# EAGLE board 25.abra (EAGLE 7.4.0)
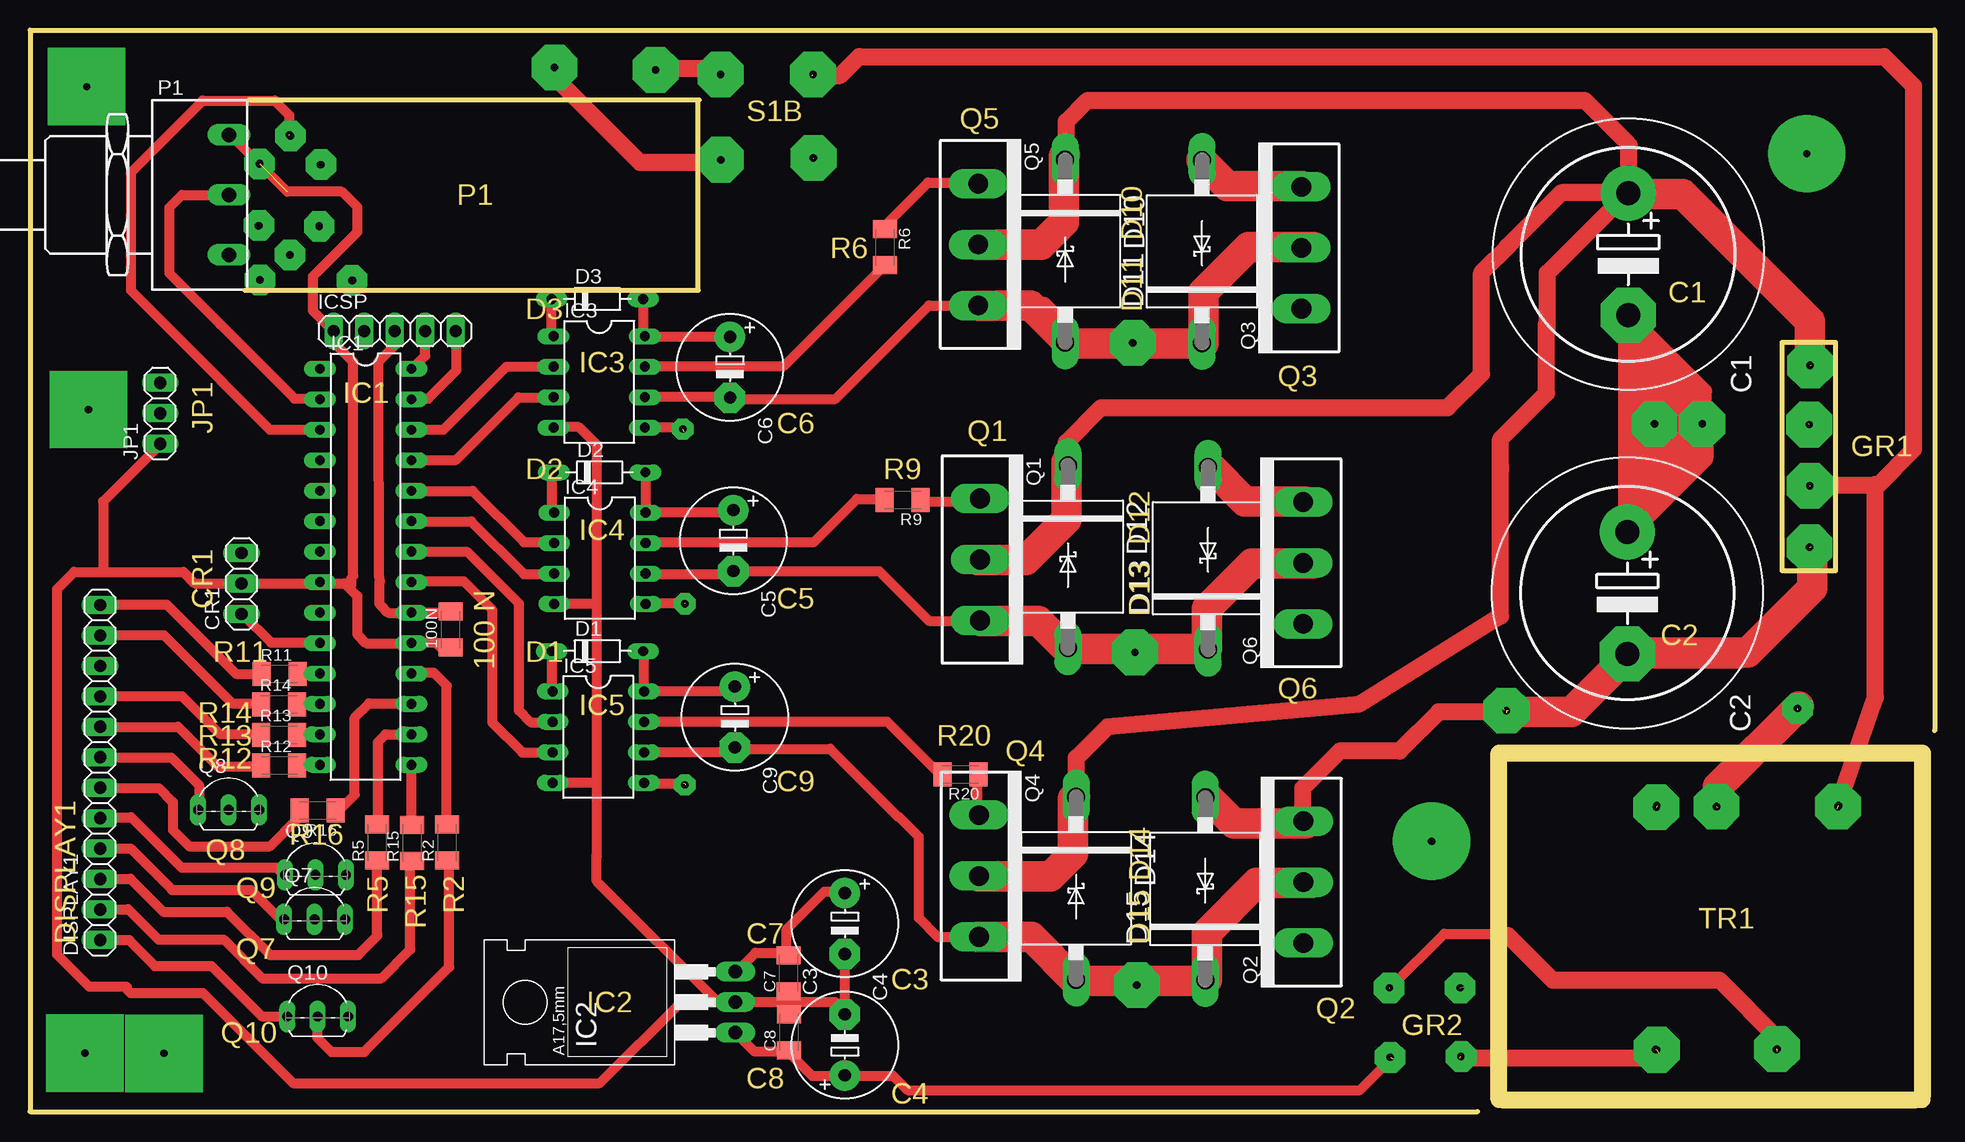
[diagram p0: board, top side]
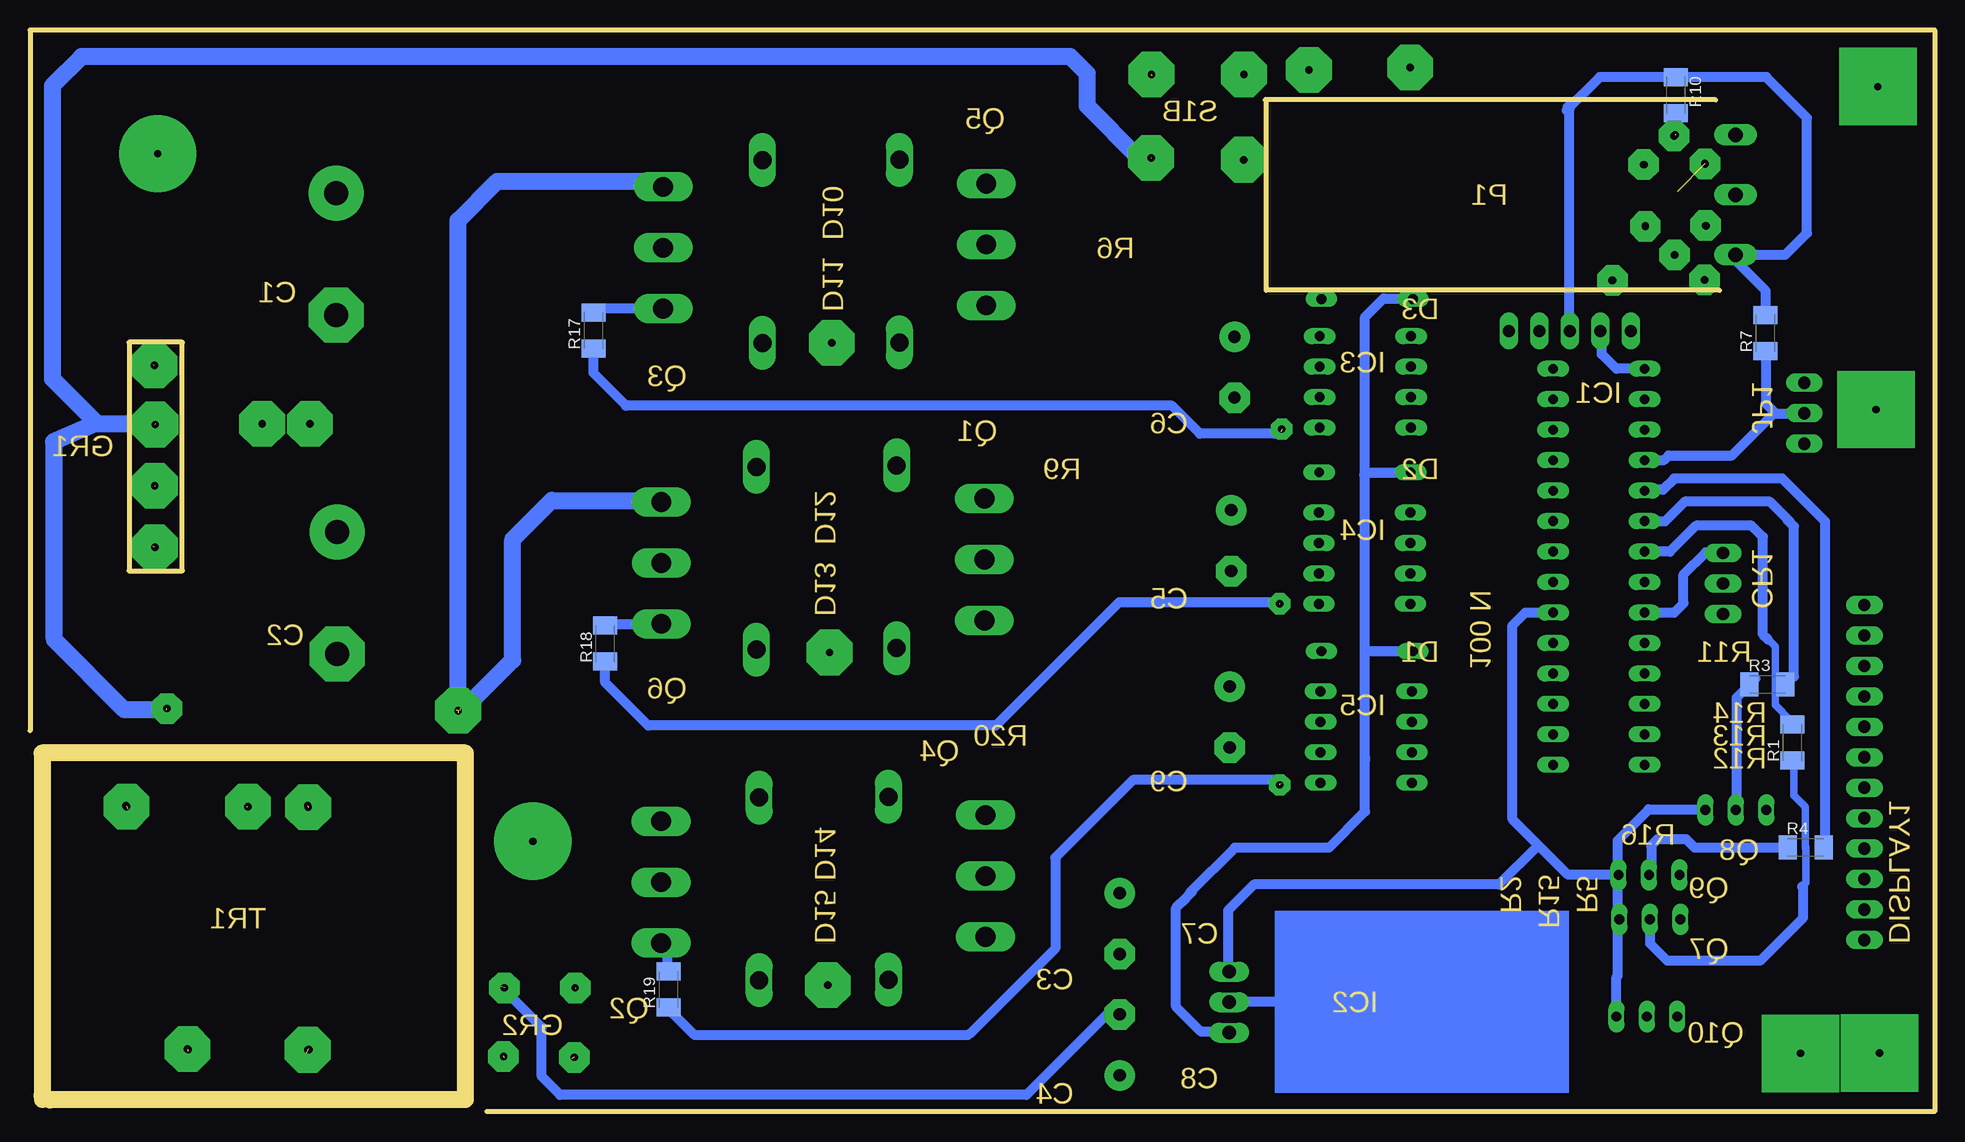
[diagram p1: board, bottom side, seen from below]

Size 158.75 x 90.17 mm. Coordinates in mm from the lower left corner, seen from the top.
Outline: 122.45,0.99 122.45,29.9 157.73,29.9 157.73,1.32
Outline: 122.66,0.99 157.07,0.96 157.71,1.02
Outline: 17.91,68.48 55.7,68.48 55.7,84.25
Outline: 18.26,84.35 55.8,84.35
Outline: 158.75,31.75 158.75,90.17 0,90.17 0,0 120.65,0
Outline: 146.05,64.14 150.5,64.14 150.5,45.09 146.05,45.09 146.05,64.14
Copper layers (1*16): Top 0.035mm / dielectric 1.5mm / Bottom 0.035mm
Design rules "default": minimum track width 10mil, minimum drill 24mil, track to track 8mil, track to pad 8mil, pad to pad 8mil, via to via 8mil, smd to smd 8mil, copper to edge 40mil, drill to drill 8mil, minimum pad ring 10mil, minimum via ring 8mil, stop-mask expansion 4mil, vias tented up to drill 0mil, thermal gap 10mil

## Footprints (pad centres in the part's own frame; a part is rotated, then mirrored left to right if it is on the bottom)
C1206K = smd 1.5 x 2: 1 -1.5,0; 2 1.5,0
EB22,5D = drill 2.007 pad 4.597: + -5.08,0 | drill 2.007 pad 4.597 octagon: - 5.08,0
E5-8,5 = drill 1.016 pad 2.54: + -2.54,0 | drill 1.016 pad 2.54 octagon: - 2.54,0
1X03 = drill 1.016 long: 1 -2.54,0; 2 0,0; 3 2.54,0
D-7.5 = drill 0.813 long: A 3.81,0; C -3.81,0
P6T15 = drill 1.499 long: A 7.62,0; C -7.62,0
1X12 = drill 1.016 long: 1 -13.97,0; 2 -11.43,0; 3 -8.89,0; 4 -6.35,0; 5 -3.81,0; 6 -1.27,0; 7 1.27,0; 8 3.81,0; 9 6.35,0; 10 8.89,0; 11 11.43,0; 12 13.97,0
DIL28-3 = drill 0.813 long: 1 -16.51,-3.81; 2 -13.97,-3.81; 3 -11.43,-3.81; 4 -8.89,-3.81; 5 -6.35,-3.81; 6 -3.81,-3.81; 7 -1.27,-3.81; 8 1.27,-3.81; 9 3.81,-3.81; 10 6.35,-3.81; 11 8.89,-3.81; 12 11.43,-3.81; 13 13.97,-3.81; 14 16.51,-3.81; 15 16.51,3.81; 16 13.97,3.81; 17 11.43,3.81; 18 8.89,3.81; 19 6.35,3.81; 20 3.81,3.81; 21 1.27,3.81; 22 -1.27,3.81; 23 -3.81,3.81; 24 -6.35,3.81; 25 -8.89,3.81; 26 -11.43,3.81; 27 -13.97,3.81; 28 -16.51,3.81
TO220 = drill 1.118 long: 1 -2.54,-10.16; 2 0,-10.16; 3 2.54,-10.16
DIL08 = drill 0.813 long: 1 -3.81,-3.81; 2 -1.27,-3.81; 3 1.27,-3.81; 4 3.81,-3.81; 5 3.81,3.81; 6 1.27,3.81; 7 -1.27,3.81; 8 -3.81,3.81
1X05 = drill 1.016 long: 1 -5.08,0; 2 -2.54,0; 3 0,0; 4 2.54,0; 5 5.08,0
PC16S = drill 1.2 long: 1A -5,6.5; 1E 5,6.5; 1S 0,6.5
TO258AA-V = drill 1.651 long: 1-D -5.08,0; 2-S 0,0; 3-G 5.08,0
TO92-BCE = drill 0.813 long: B 2.54,0; C 0,0; E -2.54,0

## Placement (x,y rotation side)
100N  [C1206K]  35.05,40.18 90 top
C1  [EB22,5D]  133.22,71.48 270 top
C2  [EB22,5D]  133.15,43.23 270 top
C3  [E5-8,5]  67.92,5.56 90 top
C4  [E5-8,5]  67.92,15.67 270 top
C5  [E5-8,5]  58.62,47.6 270 top
C6  [E5-8,5]  58.34,62.05 270 top
C7  [C1206K]  63.25,11.53 90 top
C8  [C1206K]  63.27,6.6 90 top
C9  [E5-8,5]  58.75,32.89 270 top
CR1  [1X03]  17.63,44.02 90 top
D1  [D-7.5]  47.29,38.38 0 top
D2  [D-7.5]  47.47,53.29 0 top
D3  [D-7.5]  47.29,67.74 0 top
D10  [P6T15]  86.28,71.73 270 top
D11  [P6T15]  97.69,71.7 90 top
D12  [P6T15]  86.51,46.25 270 top
D13  [P6T15]  98.2,46.13 90 top
D14  [P6T15]  87.2,18.62 270 top
D15  [P6T15]  97.97,18.57 90 top
DISPLAY1  [1X12]  5.84,28.27 90 top
IC1  [DIL28-3]  27.97,45.41 270 top
IC2  [TO220]  48.64,9.12 90 top
IC3  [DIL08]  47.45,60.83 270 top
IC4  [DIL08]  47.5,46.13 270 top
IC5  [DIL08]  47.37,31.22 270 top
ICSP  [1X05]  30.4,65.07 0 top
JP1  [1X03]  10.85,58.22 90 top
P1  [PC16S]  10.08,76.43 270 top
Q1  [TO258AA-V]  79.2,46.02 270 top
Q2  [TO258AA-V]  106.15,19.13 90 top
Q3  [TO258AA-V]  105.97,72.01 90 top
Q4  [TO258AA-V]  79.1,19.63 270 top
Q5  [TO258AA-V]  79.04,72.29 270 top
Q6  [TO258AA-V]  106.12,45.75 90 top
Q7  [TO92-BCE]  23.72,16.03 0 top
Q8  [TO92-BCE]  16.56,25.15 0 top
Q9  [TO92-BCE]  23.8,19.74 0 top
Q10  [TO92-BCE]  23.98,7.92 0 top
R1  [C1206K]  11.84,30.76 90 bottom
R2  [C1206K]  34.77,22.43 90 top
R3  [C1206K]  13.92,35.61 0 bottom
R4  [C1206K]  10.74,22.02 0 bottom
R5  [C1206K]  28.96,22.43 90 top
R6  [C1206K]  71.27,72.06 270 top
R7  [C1206K]  14.1,64.9 90 bottom
R9  [C1206K]  72.75,51 180 top
R10  [C1206K]  21.56,84.73 270 bottom
R11  [C1206K]  20.8,36.47 0 top
R12  [C1206K]  20.78,28.85 0 top
R13  [C1206K]  20.75,31.42 0 top
R14  [C1206K]  20.75,33.96 0 top
R15  [C1206K]  31.85,22.4 90 top
R16  [C1206K]  23.98,25.1 180 top
R17  [C1206K]  111.79,65.13 90 bottom
R18  [C1206K]  110.79,39.01 90 bottom
R19  [C1206K]  105.54,10.19 90 bottom
R20  [C1206K]  77.55,28.12 180 top

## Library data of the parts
100N C7 C8 Q1-Q6 R1-R7 R9-R20 = ref-packages
C1-C6 C9 = rcl
CR1 DISPLAY1 ICSP JP1 = pinhead
D1-D3 D10-D15 = diode
IC1 IC3-IC5 = 40xx
IC2 = mc33269
P1 = piher
Q7-Q10 = transistor

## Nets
S$53: ICSP.4
S$101: D1.C
S$111: Q3.2-S
S$112: D10.A
S$140: C5.-

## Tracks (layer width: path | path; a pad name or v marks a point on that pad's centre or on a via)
C5
  Top 0.813: 51.31,47.5 65.35,47.5 68.94,51.08 70.99,51.08 71.09,50.98
D1
  Top 0.813: 43.71,57.05 45.77,57.05 47.27,55.55 47.27,21.29
Q1
  Top 0.813: 79.35,77.44 74.85,77.44 71.09,73.69
S$1  (via drill 0.61 pad 6.45)
  other vias: 4.72,85.45
S$2  (via drill 0.61 pad 6.45)
  other vias: 4.57,4.88
S$3  (via drill 0.61 pad 3.81)  (1 unrouted)
  Top 1.422: 148.46,47.12 148.46,43.56 142.54,37.64 132.99,37.64 132.72,37.92
  other vias: 148.34,47.04
S$4
  Top 0.813: 5.84,42.27 11.4,42.27 17.17,36.5 18.95,36.5 19,36.45 | 19,36.45 19.15,36.45 | 19,36.45 18.41,36.45
S$5
  Top 0.813: 5.87,39.73 11.15,39.73 16.84,34.04 19.05,34.04
S$6
  Top 0.813: 5.84,34.65 12.65,34.65 15.8,31.5 18.82,31.5 18.9,31.42
S$7
  Top 0.813: 18.34,28.78 19.15,28.78
S$8
  Top 0.813: 24.16,39.09 20.09,39.09 17.65,41.53
S$9
  Bottom 0.813: 24.18,41.58 21.72,41.58 20.93,42.37 20.93,44.76 19.07,46.61 18.03,46.61 17.98,46.56
S$10
  Bottom 0.813: 34.65,4.39 34.75,4.29
S$11
  Top 0.813: 5.87,19.41 8.36,19.41 11.1,16.66 16.41,16.66 20.02,13.06 27.36,13.06 28.96,14.66
S$12
  Top 0.813: 5.84,24.54 8.43,24.54 12.62,20.34 20.55,20.34 21.29,19.61
S$13
  Top 0.813: 5.87,32.08 12.34,32.08 15.65,28.78 19.28,28.78
S$14
  Top 0.813: 5.77,14.28 8.28,14.28 10.03,12.52
S$15
  Top 0.813: 5.87,29.52 11.79,29.52 14.1,27.2 14.1,25.22 13.99,25.12
S$16
  Top 0.813: 5.82,26.98 10.72,26.98 11.91,25.78 11.91,23.47 13.26,22.12 20.02,22.12 22.28,24.38
S$17
  Top 0.813: 31.83,34.04 28.27,34.04 27.08,32.84 27.08,26.42 25.78,25.12
S$18
  Top 0.813: 31.83,31.45 29.64,31.45 29.01,30.81 29.01,23.93
S$19
  Top 0.813: 31.83,28.96 31.83,23.8 31.88,23.75
S$20
  Top 0.813: 34.75,23.98 34.75,35.51 33.68,36.58 31.95,36.58 31.77,36.4
S$21
  Top 0.813: 5.77,21.92 8.38,21.92 11.84,18.47 18.41,18.47 20.88,16
S$22
  Top 0.813: 29.06,20.78 28.96,20.68 28.96,14.78
S$23
  Top 0.813: 5.87,16.87 8.18,16.87 10.69,14.35 16.13,14.35 19.36,11.12 29.31,11.12 31.7,13.51
S$24
  Top 0.813: 31.77,20.42 31.7,20.34 31.7,13.54
S$25
  Top 0.813: 21.44,7.95 19.3,7.95 15.11,12.14 10.39,12.14 9.98,12.55
S$26
  Top 0.813: 23.98,7.95 23.98,6.12 25.12,4.98 27.86,4.98 34.95,12.06 34.95,20.5 34.52,20.93
S$27
  Top 0.813: 58.88,9.12 54.25,9.12 47.5,2.36 21.92,2.36 14.4,9.88 8.36,9.88 7.8,10.44 | 17.6,44.04 13.74,44.04 12.8,44.98 3.68,44.98 2.26,43.56 2.26,13.08 4.9,10.44 7.8,10.44 | 17.6,44.04 17.68,44.04 | 7.8,10.44 8,10.44 8.08,10.36 | 31.8,39.04 28.04,39.04 27.28,39.8 27.28,43 26.24,44.04 24.18,44.04 | 24.18,44.04 23.98,44.04 | 17.6,44.04 24.18,44.04
S$28
  Top 0.813: 31.7,39.12 33.81,39.12 34.27,38.66
S$29
  Top 0.813: 17.42,46.63 17.45,46.66
S$30
  Bottom 0.813: 31.85,41.6 34.11,41.6 35.18,40.54 35.18,24.36 30.56,19.74 26.52,19.74 26.42,19.84 | 19.13,25.2 23.82,25.2 26.42,22.61 26.42,19.84 | 26.67,7.72 26.52,7.87 26.52,11.2 26.42,11.3 26.42,19.84
S$31
  Bottom 0.813: 52.81,9.14 58.9,9.14
S$32  (via drill 0.61 pad 6.45)
  other vias: 11.18,4.85
S$33
  Top 0.813: 58.85,9.14 63.2,9.14 | 63.2,9.14 63.93,9.14 | 63.2,9.14 67.13,9.14 68.22,8.05
S$34
  Top 0.813: 63.32,5.03 60.35,5.03 58.78,6.6
S$35
  Top 0.813: 63.25,13.23 60.48,13.23 58.95,11.71
S$36
  Top 0.813: 67.92,7.92 67.92,13.11
S$37
  Top 0.813: 67.92,2.97 65.2,2.97 63.32,4.85
S$38
  Top 0.813: 67.92,18.34 66.22,18.34 63.07,15.19 63.07,13.61 63.32,13.36
S$39
  Bottom 0.813: 58.88,11.58 58.88,16.76 56.72,18.92 36.3,18.92 33.2,22.02
S$40
  Bottom 0.813: 24.56,43.99 24.51,44.04 24.28,44.04 24.36,44.12
S$41
  Bottom 0.813: 12.39,22 19.99,22 20.7,22.71 23.09,22.71 23.62,22.17 23.62,19.66 23.8,19.48
S$42
  Top 0.813: 31.7,41.6 34.8,41.6
S$43
  Bottom 0.813: 24.16,46.69 22.05,46.69 19.89,48.84 15.27,48.84 14.33,47.9
S$44
  Bottom 0.813: 24.21,49.2 22.48,49.2 20.83,50.85 13.74,50.85 11.99,49.1
S$45
  Bottom 0.813: 24.21,51.84 22.63,51.84 21.69,52.78 12.7,52.78 9.12,49.2 9.12,46.46 | 9.12,22.05 9.12,46.46 | 9.12,46.46 9.12,46.69
S$46
  Bottom 0.813: 16.48,25.15 16.48,34.52 14.91,36.09
S$47
  Bottom 0.813: 11.71,36.27 11.71,48.79 12.29,49.38
S$48
  Bottom 0.813: 23.7,16.08 23.7,13.99 22.28,12.57 14.53,12.57 10.95,16.15 10.95,18.67 11.05,18.77
S$49
  Bottom 0.61: 10.77,22 10.77,25.4 11.71,26.34 11.71,28.8 11.81,28.91
S$50
  Bottom 0.61: 10.74,22.07 10.74,19.05 11.02,18.77
S$51
  Bottom 0.61: 13.28,37.03 13.28,37.06 | 13.28,37.03 13.28,33.88 11.96,32.56 | 13.28,37.03 13.28,38.79 14.05,39.55
S$52
  Bottom 0.813: 14.3,47.93 14.3,39.78 13.87,39.34
S$53
  Top 0.813: ICSP.4 32.94,63.02 31.77,61.85
S$54
  Top 0.813: 31.65,59.44 33.2,59.44 35.56,61.8 35.56,65.05 35.43,65.18
S$55
  Top 0.813: 31.95,59.46 31.85,59.36
S$56
  Top 0.813: 31.8,41.58 29.87,41.58 29.13,42.32 29.13,44.15
S$57
  Top 0.813: 29.08,60.55 29.11,44.53 29.16,44.17
S$58
  Bottom 0.813: 24.36,44.17 24.31,44.12
S$59
  Top 0.813: 26.77,43.92 26.77,44.48 26.95,44.65 26.95,62.48 25.2,64.24
S$60  (via drill 0.61 pad 1.78, 0.61 pad 2.54)  (2 unrouted)
  Top 0.813: 21.61,81.38 21.61,83.06 20.4,84.28 14.38,84.28 8.43,78.33 8.43,68.45 16.05,60.83
  Bottom 0.813: 21.57,83.08 21.57,81.46 21.54,81.43
  other vias: 21.62,81.43 21.72,81.33
S$61  (via drill 0.61 pad 1.78, 0.61 pad 2.54)
  other vias: 21.67,71.4 21.67,71.42
S$62  (via drill 0.61 pad 1.78, 0.61 pad 2.54)
  other vias: 19.18,69.32 19.18,69.34
S$63  (via drill 0.61 pad 1.78, 0.61 pad 2.54)  (1 unrouted)
  Top 0.813: 16.56,81.43 16.69,81.43 v19.13,78.99 21.44,76.68 26.01,76.68 27.3,75.39 27.3,73.36 23.6,69.65 23.6,66.75 25.38,64.97
  other vias: 19.15,79.04
S$64  (via drill 0.61 pad 1.78, 0.61 pad 2.54)
  other vias: 24.21,78.94 24.26,78.94
S$65  (via drill 0.61 pad 1.78, 0.61 pad 2.54)
  other vias: 24.1,73.84 24.1,73.79
S$66  (via drill 0.61 pad 1.78, 0.61 pad 2.54)
  other vias: 19.05,73.84 19.1,73.86
S$67  (via drill 0.61 pad 1.78, 0.61 pad 2.54)
  other vias: 26.9,69.29 26.82,69.29
S$68
  Top 0.813: 16.66,76.4 12.65,76.4 11.63,75.39 11.63,69.88 15.85,65.66 15.85,65.63 22.05,59.44 24.11,59.44 24.31,59.23
S$69
  Bottom 0.813: 24.21,61.92 26.52,61.92 27.74,63.14 27.74,64.9 27.91,65.08
S$70
  Bottom 0.813: 30.43,65.2 30.43,83.62 30.58,83.77
S$71
  Top 0.813: 29.06,60.55 29.06,62.53 30.68,64.16
S$72
  Top 0.813: 16.59,76.78 16.97,76.4
S$73
  Top 0.813: 24.16,56.84 19.99,56.84 15.9,60.94
S$74
  Bottom 0.813: 30.68,83.46 27.91,86.23 14.02,86.23 10.64,82.86 10.64,73.23 12.47,71.4 16.61,71.4
S$75
  Bottom 0.813: 30.35,65.08 30.68,65.41
S$76
  Top 0.813: 31.8,56.84 34.47,56.84 39.73,62.1 43.43,62.1 43.48,62.05
S$77
  Top 0.813: 31.75,54.33 35.51,54.33 40.72,59.54 43.51,59.54 43.56,59.59
S$78
  Top 0.813: 32.21,51.97 31.98,51.74
S$79
  Top 0.813: 31.8,51.74 36.91,51.74 41.17,47.47 43.94,47.47 43.99,47.42
S$80
  Top 0.813: 43.54,32.41 43.48,32.46
S$81
  Top 0.813: 31.8,49.2 36.78,49.2 41.17,44.81 43.84,44.81 43.94,44.7
S$82
  Top 0.813: 31.75,46.63 36.5,46.63 40.77,42.37 40.77,33.43 41.73,32.46 43.56,32.46 43.61,32.41
S$83
  Top 0.813: 31.7,44.2 36.17,44.2 38.56,41.81 38.56,32.41 41.05,29.92 43.81,29.92 43.87,29.87
S$84
  Top 0.813: 43.71,44.78 43.66,44.83
S$86
  Top 0.813: 43.56,27.43 47.19,27.43
S$87
  Top 0.813: 43.71,42.37 47.19,42.37 47.24,42.42
S$88
  Top 0.813: 47.24,21.49 47.24,19.2 57.35,9.09
S$89
  Top 0.813: 43.54,38.43 43.54,35.15 43.61,35.08
S$90
  Top 0.813: 51.18,34.9 51.18,38.33
S$91
  Top 0.813: 51.13,67.69 51.13,64.92 51.41,64.64
S$92
  Top 0.813: 51.36,53.39 51.36,50.01 51.31,49.96
S$93
  Top 0.813: 43.54,53.39 43.54,49.94 43.66,49.81
S$94
  Top 0.813: 43.48,67.84 43.48,64.95 43.89,64.54
S$95
  Top 0.813: 51.31,64.59 58.5,64.59
S$96
  Top 0.813: 51.18,59.59 58.47,59.59 58.62,59.44
S$97
  Top 0.813: 51.26,49.96 58.73,49.96 58.78,50.01
S$98
  Top 0.813: 51.31,44.81 58.29,44.81 58.62,45.14
S$99
  Top 0.813: 51.13,35.08 59.05,35.08 59.16,35.18
S$100
  Top 0.813: 51.21,29.97 58.67,29.97 58.83,30.12
S$101
  Bottom 0.813: 43.41,67.79 45.92,67.79 47.47,66.24 47.47,38.51 | D1.C 47.35,38.38 47.47,38.51 | 47.47,29.49 47.47,38.51 | 47.47,29.49 47.47,29.29 | 47.47,29.49 47.47,25.02 50.49,22 58.32,22 62.1,18.21
S$102
  Bottom 0.813: 43.69,53.24 47.4,53.24 47.55,53.09
S$103  (via drill 0.61 pad 3.81)  (2 unrouted)
  Top 1.422: 65.18,86.36 67.51,86.36 69.11,87.96 154.56,87.96 157,85.52 157,55.19 154,52.2 148.46,52.2 148.36,52.09
  other vias: 65.28,86.46 148.36,52.17
S$104  (via drill 0.61 pad 3.81)  (2 unrouted)
  Bottom 1.422: 65.28,79.5 66.29,79.5 70.61,83.82 70.61,86.54 72.03,87.96 154.46,87.96 156.9,85.52 156.9,61.09 153.16,57.35 148.28,57.35 148.18,57.25
  other vias: 65.3,79.5 148.31,57.28
S$105
  Bottom 1.422: 156.79,55.85 153.34,57.35
S$106  (via drill 0.61 pad 3.81)
  other vias: 57.56,86.46
S$107
  Bottom 0.813: 24.21,54.33 22.53,54.33 22.15,54.71 16.89,54.71 13.41,58.19 13.23,58.19 | 13.23,58.19 10.79,58.19 | 14.07,63.35 14.07,59.03 13.23,58.19
S$108
  Top 1.422: 79.15,72.29 84.58,72.29 86.18,73.89 86.18,74.14 86.18,79.15 86.46,79.43
  Top 2.54: 78.87,72.26 84.3,72.26 86.18,74.14 86.18,79.65 86.28,79.76
S$109
  Top 1.422: 79.15,67.21 84.51,67.21 86.39,65.33 86.39,64.03 86.28,63.93
S$110
  Top 1.422: 105.89,77.27 99.77,77.27 97.81,79.22
S$111
  Top 1.422: Q3.2-S 101.68,72.01 97.71,68.05 97.71,64.31 97.81,64.21
S$112
  Top 1.422: D10.A 97.71,64.11
S$113  (via drill 0.61 pad 3.81)  (1 unrouted)
  Top 1.422: 133.27,76.4 133.27,76.48 133.27,76.61 | 133.27,76.61 133.27,80.59 133.17,80.7 | 133.27,76.61 127.64,76.61 123.14,72.11 | 141.63,72.67 148.46,65.84 148.46,62.23
  Top 2.54: 133.27,76.48 137.77,76.48 148.36,65.89 148.36,62.41 148.18,62.23
  other vias: 148.39,62.2
S$114
  Top 1.422: 133.17,80.72 129.59,84.3 88.16,84.3 86.39,82.53 86.39,79.15
S$115
  Top 1.422: 79.15,45.9 82.88,45.9 86.46,49.48 86.46,53.77 86.56,53.87
S$116
  Top 1.422: 79.15,40.84 84.2,40.84 86.56,38.48 98.09,38.48 98.37,38.2 98.37,42.42 101.58,45.62 106.63,45.62 106.83,45.82
S$117
  Top 1.422: 106.07,50.88 100.91,50.88 98.09,53.7
S$118  (via drill 0.61 pad 2.54, 0.61 pad 3.81)  (2 unrouted)
  Top 1.422: 145.62,4.55 145.62,5.03
  other vias: 145.62,5.21 145.57,5.18
S$119  (via drill 0.61 pad 3.81)  (3 unrouted)
  Top 1.422: 133.27,38.12 128.57,33.43 123.22,33.43 122.89,33.43 | 122.86,33.6 122.86,33.12 | 123.14,33.33 117.42,33.33 114.15,30.05 109.17,30.05 106.07,26.95 106.07,23.93 106.25,23.75
  Top 2.54: 123.14,33.33 128.5,33.33 133.45,38.28 143.21,38.28 148.56,43.64 148.56,46.46 148.74,46.63
  Bottom 1.422: 105.54,77.55 119.81,77.55 123.06,74.3 123.06,33.25
  other vias: 123.06,33.43
S$120
  Top 1.422: 79.15,19.53 84.89,19.53 87.05,21.69 87.05,26.11 87.22,26.29 | 87.22,26.29 87.4,26.47 | 87.22,26.29 87.22,29.49 89.84,32.11 110.85,33.98 122.58,41.3 122.58,53.52 | 122.58,53.52 122.58,53.8 | 122.58,53.52 122.58,56.06 126.42,59.89 126.42,65.71
S$121
  Bottom 0.813: 14.07,66.45 14.07,68.43 16.79,71.14
S$122
  Top 1.422: 106.25,24.03 100.08,24.03 98.02,26.09
S$123
  Bottom 1.422: 106.05,50.95 115.27,50.95 118.52,47.7 118.52,37.64 122.73,33.43
S$124  (via drill 0.61 pad 3.81)
  other vias: 92.1,38.28
S$125  (via drill 0.61 pad 3.81)
  other vias: 92.25,10.54
S$126  (via drill 0.61 pad 3.81)
  other vias: 91.92,64.08
S$128
  Top 0.813: 50.83,62.15 62.84,62.15 71.09,70.41
S$129
  Top 0.813: 58.42,59.41 67.13,59.41 74.93,67.21 78.77,67.21 78.87,67.11
S$130
  Bottom 0.813: 106.07,66.93 111.33,66.93 111.61,66.65
S$131
  Bottom 0.813: 111.78,63.55 111.78,61.57 109.07,58.85 63.58,58.85 61.24,56.52 54.97,56.52 54.41,57.07
S$132  (via drill 0.61 pad 1.78)  (1 unrouted)
  Top 0.813: 51.31,57.07 54.1,57.07 54.48,56.69
  other vias: 54.41,56.9
S$133
  Top 0.813: 79.05,14.55 78.97,14.55 75.67,14.55 74.09,16.13 74.09,22.91 72.47,24.54
  Top 1.422: 79.15,14.66 83.36,14.66 87.12,10.9 98.2,10.9 98.2,15.49 101.85,19.15 106.07,19.15 106.25,18.97
  Top 2.54: 78.97,14.55 83.46,14.55 87.12,10.9 98.02,10.9 98.09,10.97 98.09,14.91 102.23,19.05 106.91,19.05
S$134  (via drill 0.61 pad 6.45)
  other vias: 148.11,79.86
S$135
  Top 0.813: 78.97,24.79 78.97,28.07 79.07,28.17
S$136
  Top 0.813: 78.97,50.88 74.37,50.88 74.27,50.98
S$137
  Bottom 0.813: 58.75,6.58 58.67,6.5
S$138
  Bottom 0.813: 58.9,6.66 61.14,6.66 63.22,8.74 63.22,16.97 62.36,17.83
S$140
  Top 0.813: C5.- 70.79,45.06 74.93,40.92 78.89,40.92 78.97,40.84
S$141
  Bottom 0.813: 106.02,40.62 110.41,40.62 110.52,40.51
S$142  (via drill 0.61 pad 1.78)  (2 unrouted)
  Top 0.813: 51.31,42.39 54.51,42.39 54.56,42.34
  Bottom 0.813: 110.8,37.47 110.8,35.76 107.21,32.18 78.23,32.18 67.97,42.44 54.71,42.44 54.61,42.34
  other vias: 54.58,42.34
S$143
  Top 0.813: 51.18,32.51 71.45,32.51 75.84,28.12
S$144
  Top 0.813: 72.42,24.54 66.7,30.25 58.73,30.25
S$145
  Top 0.813: 79.2,14.38 78.92,14.66
S$146
  Bottom 0.813: 62.36,17.86 61.9,18.31
S$147  (via drill 0.61 pad 1.78)  (2 unrouted)
  Top 0.813: 54.71,27.1 54.46,27.36 51.13,27.36
  Bottom 0.813: 80.44,6.45 73.28,13.61 73.28,21.18 66.83,27.64 54.94,27.64 54.61,27.3
  other vias: 54.58,27.23
S$148  (via drill 0.61 pad 6.45)
  other vias: 116.84,22.53
S$149  (via drill 0.61 pad 2.54, 0.61 pad 3.81)  (3 unrouted)
  Top 1.422: 119.2,4.5 135.33,4.5 135.71,4.88
  other vias: 119.28,4.6 135.51,5.18 135.61,5.16
S$150  (via drill 0.61 pad 2.54)  (1 unrouted)
  Top 0.813: 113.39,10.24 113.39,10.34 117.88,14.83 122.86,14.83 123.9,13.79
  Top 1.422: 113.28,10.24 113.28,10.52
  other vias: 113.31,10.31
S$151
  Top 1.422: 145.75,6.02 140.79,10.97 126.9,10.97 123.22,14.66
S$152
  Bottom 0.813: 105.61,11.63 105.61,13.44 106.07,13.89
S$153
  Bottom 0.813: 80.57,6.38 103.35,6.38 105.51,8.53
S$154  (via drill 0.61 pad 2.54)  (1 unrouted)
  Bottom 0.813: 67.89,8.08 69.01,8.08 75.69,1.4 114.58,1.4 116.1,2.92 116.1,7.04 119.48,10.41
  other vias: 119.2,10.31
S$155  (via drill 0.61 pad 2.54, 0.61 pad 3.81)  (3 unrouted)
  Top 1.422: 140.69,25.35 140.69,25.53 140.69,26.95 v147.34,33.6
  Top 2.54: 140.69,25.53 140.69,27.05 147.42,33.78
  Bottom 1.422: 147.34,33.5 150.88,33.5 156.72,39.34 156.72,55.68 156.44,55.96
  other vias: 140.59,25.4 140.59,25.43
S$156  (via drill 0.61 pad 2.54)  (1 unrouted)
  Top 0.813: 67.89,3 71.93,3 73.15,1.78 110.85,1.78 113.49,4.42
  other vias: 113.39,4.52
S$157  (via drill 0.61 pad 6.45)
  other vias: 4.88,58.52
S$158  (via drill 0.61 pad 3.81)
  Top 1.422: 52.12,86.97 57.56,86.97 57.76,86.77
  other vias: 52.15,86.84
S$159  (via drill 0.61 pad 3.81)
  Top 1.422: 43.76,86.97 43.76,86.21 50.83,79.15 57.45,79.15
  other vias: 43.71,87.05 57.58,79.35
S$160
  Top 1.422: 133.27,76.3 138.05,76.3 142.32,72.03
S$161
  Top 1.422: 126.47,65.2 126.47,69.9 133.35,76.78
S$162
  Top 1.422: 133.07,66.37 133.07,48.18 133.17,48.08
S$163  (via drill 0.61 pad 3.81)
  Top 1.422: 139.6,57.23 139.6,54.43 133.35,48.18 | 139.5,57.53 139.5,60.05 133.17,66.37
  other vias: 139.4,57.33
S$164  (via drill 0.61 pad 3.81)
  other vias: 135.41,57.33
S$165
  Top 2.54: 133.86,64.34 133.86,51.1 | 133.86,50.52 133.86,51.1 | 133.86,51.1 138.02,55.27 138.02,59.46 135.2,62.28 135.2,54.89 135.69,54.41 135.69,58.09 136.47,58.88
S$166
  Top 2.54: 106.25,50.88 101.27,50.88 98.48,53.67
S$167
  Top 1.422: 123.34,72.29 120.98,69.93 120.98,61.49 118.16,58.67 89.28,58.67 86.39,55.78 86.39,54.15 86.39,53.59
  Top 2.54: 78.97,45.97 83.01,45.97 86.39,49.35 86.39,54.15
S$168
  Top 2.54: 79.25,40.92 84.05,40.92 86.39,38.58 98.09,38.58 98.09,41.94 101.85,45.7 106.91,45.7
S$169  (via drill 0.61 pad 2.54, 0.61 pad 3.81)  (2 unrouted)
  Top 1.422: 153.82,52.3 153.82,34.54 150.62,25.25
  other vias: 150.75,25.5 150.7,25.43
S$170
  Top 2.54: 79.07,19.61 85.06,19.61 86.94,21.49 86.94,26.11 87.12,26.29
S$171
  Top 2.54: 106.35,24.03 100.36,24.03 98.2,26.19
S$172
  Top 2.54: 79.07,67.18 83.39,67.18 86.56,64.01 97.81,64.01 97.81,68.33 101.58,72.08 107.01,72.08
S$173
  Top 2.54: 106.07,77.14 99.8,77.14 97.64,79.3
S$174
  Top 0.813: 10.79,55.65 10.79,55.58 6.1,50.88 6.1,45.24
S$178  (via drill 0.61 pad 2.54, 0.61 pad 3.81)  (1 unrouted)
  other vias: 135.61,25.5 135.56,25.37
(copper drawn outside any net)
  shapes: Bottom area x1

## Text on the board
Dimension: S1B | Q5 | P1 | R6 | C1 | D11 D10 | D3 | IC3 | Q3 | IC1 | JP1 | C6 | Q1 | GR1 | D2 | R9 | IC4 | CR1 | C5 | D13 D12 | C2 | R11 | 100 N | D1 | Q6 | IC5 | R14 | R13 | R20 | R12 | Q4 | C9 | R16 | Q8 | Q9 | R5 | R2 | R15 | TR1 | DISPLAY1 | C7 | D15 D14 | Q7 | C3 | Q2 | IC2 | Q10 | GR2 | C8 | C4
101: R10 | R7 | R17 | R18 | R3 | R1 | R4 | R19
